| TEXAS INSTRUMENTS INCORPORATED
| Standard Linear and Logic Group
| IBIS Model of SN74LVC2G53
| Single-pole double-throw (SPDT) analog switch or 2:1 analog
| muliplexer/demultiplexer
| This file contains package information for the following:
|  SOT 8-pin (DCT) package as [Component] LVC2G53_DCT
|  DSBGA 8-pin (YEP_YZP) package as [Component] LVC2G53_YEP_YZP
|  DSBGA 8-pin (YEA_YZA) package as [Component] LVC2G53_YEA_YZA
|  SOT 8-pin (DCU) package as [Component] LVC2G53_DCU
| This device can be powered at the following Vccs:
|  1.8 volt Vcc
|  2.5 volt Vcc
|  3.3 volt Vcc
|  5 volt Vcc
| This file provides unique models under the [Model Selector] for each Vcc.
| For operation at a specific Vcc, select the appropriate model after each
| [Model Selector] keyword.
[IBIS Ver]   3.2
[Comment char]  |_char
[File Name]   sn74lvc2g53.ibs
[File Rev]   1.1 | x_die
[Date]   January 10, 2005
[Source]   Data created from TI-SPICE simulations at TI-SLL.
[Notes]   The following is an IBIS list for the LVC2G53.
   Please contact sllibis@ti.com with questions and
   comments concerning SLL IBIS models.
   - FILE REV HISTORY
   - 1.1 Release IBIS file on 01/26/05
   - Power clamp data deleted in the INH and A models as there
   is no power-clamp diode.
   - Non-monotonic data due to FET characteristics.
   - NCH & PCH MOSFETS, so [Series Mosfet] model can have rising
   or falling currents
[Disclaimer] Property of Texas Instruments Incorporated.  Unauthorized
   reproduction and/or distribution is strictly prohibited.
   This product is protected under copyright law.
   Created  2005, (C) Copyright  2005, Texas Instruments
   Incorporated, All Rights Reserved
   UNLESS THERE IS A SIGNED, WRITTEN AGREEMENT TO THE
   CONTRARY, TEXAS INSTRUMENTS (TI) IS PROVIDING THE IBIS
   MODELS  AND WITHOUT ANY WARRANTY, EXPRESSED OR
   IMPLIED.  TI assumes no liability for:
   1) the accuracy of the IBIS models provided to your
   company;
   2) the proper functioning of these IBIS Models in your
   design or for any resulting applications; or
   3) infringement of patents, copyrights or intellectual
   property rights resulting from your use of these IBIS
   models.
   TI provides IBIS Models as a service to our customers.
   You and your company shall not distribute, sell or give
   these models to anyone else without prior written
   permission from TI.
   TI reserves the right to make changes to our products or
   to discontinue any semiconductor product or service
   without notice, and advises our customers to obtain the
   latest version of relevant information to verify, before
   placing orders, that the information being relied on is
   current.
   Please be aware that your receipt and use of the IBIS
   information provided shall serve as acceptance of these
   terms and conditions.  If you do not accept these terms,
   you should return or destroy the IBIS models and any
   other accompanying information immediately.
| Component LVC2G53_DCT 8-pin SOT
[Component]   LVC2G53_DCT
[Manufacturer]   Texas Instruments, Inc.
[Package]
|   typ   min   max
R_pkg   2.900e-02   2.800e-02   3.100e-02
L_pkg   1.796e-09   1.666e-09   1.924e-09
C_pkg   2.310e-13   2.210e-13   2.420e-13
[Pin]   signal_name   model_name   R_pin   L_pin   C_pin
1   COM   LVC2G53_COM   3.100e-02   1.894e-09   2.230e-13
2   INH   LVC2G53_INH   2.800e-02   1.697e-09   2.370e-13
3   GND   GND   3.000e-02   1.722e-09   2.390e-13
4   GND   GND   3.000e-02   1.861e-09   2.210e-13
5   A   LVC2G53_A   2.800e-02   1.924e-09   2.280e-13
6   Y2   LVC2G53_Y   2.900e-02   1.736e-09   2.420e-13
7   Y1   LVC2G53_Y   2.800e-02   1.666e-09   2.360e-13
8   VCC   POWER   3.000e-02   1.871e-09   2.220e-13
| Component LVC2G53_YEP_YZP 8-pin DSBGA
[Component]   LVC2G53_YEP_YZP
[Manufacturer]   Texas Instruments, Inc.
[Package]
|   typ   min   max
R_pkg   1.000e-03   1.000e-03   4.000e-03
L_pkg   6.400e-11   2.400e-11   3.790e-10
C_pkg   5.800e-14   0.000e+00   6.700e-14
[Pin]   signal_name   model_name   R_pin   L_pin   C_pin
1   COM   LVC2G53_COM   1.000e-03   2.500e-11   6.400e-14
2   INH   LVC2G53_INH   1.000e-03   2.400e-11   6.700e-14
3   GND   GND   1.000e-03   2.400e-11   6.700e-14
4   GND   GND   1.000e-03   2.500e-11   6.400e-14
5   A   LVC2G53_A   1.000e-03   2.500e-11   6.400e-14
6   Y2   LVC2G53_Y   1.000e-03   2.400e-11   6.700e-14
7   Y1   LVC2G53_Y   1.000e-03   2.400e-11   6.700e-14
8   VCC   POWER   1.000e-03   2.500e-11   6.400e-14
| Component LVC2G53_YEA_YZA 8-pin DSBGA
[Component]   LVC2G53_YEA_YZA
[Manufacturer]   Texas Instruments, Inc.
[Package]
|   typ   min   max
R_pkg   1.000e-03   1.000e-03   1.000e-03
L_pkg   2.100e-11   2.100e-11   2.100e-11
C_pkg   4.300e-14   4.200e-14   4.400e-14
[Pin]   signal_name   model_name   R_pin   L_pin   C_pin
1   COM   LVC2G53_COM   1.000e-03   2.100e-11   4.300e-14
2   INH   LVC2G53_INH   1.000e-03   2.100e-11   4.400e-14
3   GND   GND   1.000e-03   2.100e-11   4.400e-14
4   GND   GND   1.000e-03   2.100e-11   4.300e-14
5   A   LVC2G53_A   1.000e-03   2.100e-11   4.200e-14
6   Y2   LVC2G53_Y   1.000e-03   2.100e-11   4.300e-14
7   Y1   LVC2G53_Y   1.000e-03   2.100e-11   4.300e-14
8   VCC   POWER   1.000e-03   2.100e-11   4.200e-14
| Component LVC2G53_DCU 8-pin SOT
[Component]   LVC2G53_DCU
[Manufacturer]   Texas Instruments, Inc.
[Package]
|   typ   min   max
R_pkg   2.600e-02   2.300e-02   3.800e-02
L_pkg   1.394e-09   1.066e-09   2.046e-09
C_pkg   2.590e-13   2.150e-13   3.720e-13
[Pin]   signal_name   model_name   R_pin   L_pin   C_pin
1   COM   LVC2G53_COM   2.400e-02   1.520e-09   2.710e-13
2   INH   LVC2G53_INH   2.300e-02   1.112e-09   2.180e-13
3   GND   GND   2.300e-02   1.070e-09   2.170e-13
4   GND   GND   2.700e-02   2.046e-09   3.720e-13
5   A   LVC2G53_A   2.700e-02   1.542e-09   2.730e-13
6   Y2   LVC2G53_Y   2.300e-02   1.100e-09   2.240e-13
7   Y1   LVC2G53_Y   2.300e-02   1.066e-09   2.150e-13
8   VCC   POWER   3.800e-02   1.696e-09   2.800e-13
[Series Switch Groups]
| Function Group States
On  1 /   | COM->Y1 INH LOW, A LOW
On  2 /   | COM->Y2 INH LOW, A HIGH
On  3 /   | Y1->COM INH LOW, A LOW
On  4 /   | Y2->COM INH LOW, A HIGH
Off 1 2 3 4 /   | INH HIGH
[Series Pin Mapping]   pin_2   model_name   function_table_group
1   7   LVC2G53_COM_18_S   1
| 1   7   LVC2G53_COM_25_S   1
| 1   7   LVC2G53_COM_33_S   1
| 1   7   LVC2G53_COM_50_S   1
1   6   LVC2G53_COM_18_S   2
| 1   6   LVC2G53_COM_25_S   2
| 1   6   LVC2G53_COM_33_S   2
| 1   6   LVC2G53_COM_50_S   2
7   1   LVC2G53_Y_18_S   3
| 7   1   LVC2G53_Y_25_S   3
| 7   1   LVC2G53_Y_33_S   3
| 7   1   LVC2G53_Y_50_S   3
6   1   LVC2G53_Y_18_S   4
| 6   1   LVC2G53_Y_25_S   4
| 6   1   LVC2G53_Y_33_S   4
| 6   1   LVC2G53_Y_50_S   4
| Model LVC2G53_INH
[Model Selector]   LVC2G53_INH
LVC2G53_INH_18   1.8 volt Vcc
LVC2G53_INH_25   2.5 volt Vcc
LVC2G53_INH_33   3.3 volt Vcc
LVC2G53_INH_50   5 volt Vcc
| Model LVC2G53_A
[Model Selector]   LVC2G53_A
LVC2G53_A_18   1.8 volt Vcc
LVC2G53_A_25   2.5 volt Vcc
LVC2G53_A_33   3.3 volt Vcc
LVC2G53_A_50   5 volt Vcc
| Model LVC2G53_COM
[Model Selector]   LVC2G53_COM
LVC2G53_COM_18   1.8 volt Vcc
LVC2G53_COM_25   2.5 volt Vcc
LVC2G53_COM_33   3.3 volt Vcc
LVC2G53_COM_50   5 volt Vcc
| Model LVC2G53_COM_S
[Model Selector]   LVC2G53_COM_S
LVC2G53_COM_18_S   1.8 volt Vcc
LVC2G53_COM_25_S   2.5 volt Vcc
LVC2G53_COM_33_S   3.3 volt Vcc
LVC2G53_COM_50_S   5 volt Vcc
| Model LVC2G53_Y
[Model Selector]   LVC2G53_Y
LVC2G53_Y_18   1.8 volt Vcc
LVC2G53_Y_25   2.5 volt Vcc
LVC2G53_Y_33   3.3 volt Vcc
LVC2G53_Y_50   5 volt Vcc
| Model LVC2G53_Y_S
[Model Selector]   LVC2G53_Y_S
LVC2G53_Y_18_S   1.8 volt Vcc
LVC2G53_Y_25_S   2.5 volt Vcc
LVC2G53_Y_33_S   3.3 volt Vcc
LVC2G53_Y_50_S   5 volt Vcc
[Model]   LVC2G53_COM_18_S
Model_type  Series_switch
| variable   typ   min   max
C_comp   0   0   0
[Temperature Range]   40   100   -40
| Ambient temperature   25   85   -40
[Voltage range]   1.8   1.65   1.95
[On]
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[Off]
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[Model]   LVC2G53_COM_25_S
Model_type  Series_switch
| variable   typ   min   max
C_comp   0   0   0
[Temperature Range]   40   100   -40
| Ambient temperature   25   85   -40
[Voltage range]   2.5   2.3   2.7
[On]
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[Off]
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[Model]   LVC2G53_COM_33_S
Model_type  Series_switch
| variable   typ   min   max
C_comp   0   0   0
[Temperature Range]   40   100   -40
| Ambient temperature   25   85   -40
[Voltage range]   3.3   3   3.6
[On]
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[Off]
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[Model]   LVC2G53_COM_50_S
Model_type  Series_switch
| variable   typ   min   max
C_comp   0   0   0
[Temperature Range]   40   100   -40
| Ambient temperature   25   85   -40
[Voltage range]   5   4.5   5.5
[On]
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[Off]
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[Model]   LVC2G53_Y_18_S
Model_type  Series_switch
| variable   typ   min   max
C_comp   0   0   0
[Temperature Range]   40   100   -40
| Ambient temperature   25   85   -40
[Voltage range]   1.8   1.65   1.95
[On]
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[Off]
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[Model]   LVC2G53_Y_25_S
Model_type  Series_switch
| variable   typ   min   max
C_comp   0   0   0
[Temperature Range]   40   100   -40
| Ambient temperature   25   85   -40
[Voltage range]   2.5   2.3   2.7
[On]
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[Off]
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[Model]   LVC2G53_Y_33_S
Model_type  Series_switch
| variable   typ   min   max
C_comp   0   0   0
[Temperature Range]   40   100   -40
| Ambient temperature   25   85   -40
[Voltage range]   3.3   3   3.6
[On]
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[Off]
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[Model]   LVC2G53_Y_50_S
Model_type  Series_switch
| variable   typ   min   max
C_comp   0   0   0
[Temperature Range]   40   100   -40
| Ambient temperature   25   85   -40
[Voltage range]   5   4.5   5.5
[On]
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[Off]
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| Models and submodels in the file (24): LVC2G53_INH_18 (Input), LVC2G53_INH_25 (Input), LVC2G53_INH_33 (Input), LVC2G53_INH_50 (Input), LVC2G53_A_18 (Input), LVC2G53_A_25 (Input), LVC2G53_A_33 (Input), LVC2G53_A_50 (Input), LVC2G53_COM_18_S (Series_switch), LVC2G53_COM_18 (Terminator), LVC2G53_COM_25_S (Series_switch), LVC2G53_COM_25 (Terminator), LVC2G53_COM_33_S (Series_switch), LVC2G53_COM_33 (Terminator), LVC2G53_COM_50_S (Series_switch), LVC2G53_COM_50 (Terminator), LVC2G53_Y_18_S (Series_switch), LVC2G53_Y_18 (Terminator), LVC2G53_Y_25_S (Series_switch), LVC2G53_Y_25 (Terminator), LVC2G53_Y_33_S (Series_switch), LVC2G53_Y_33 (Terminator), LVC2G53_Y_50_S (Series_switch), LVC2G53_Y_50 (Terminator)
